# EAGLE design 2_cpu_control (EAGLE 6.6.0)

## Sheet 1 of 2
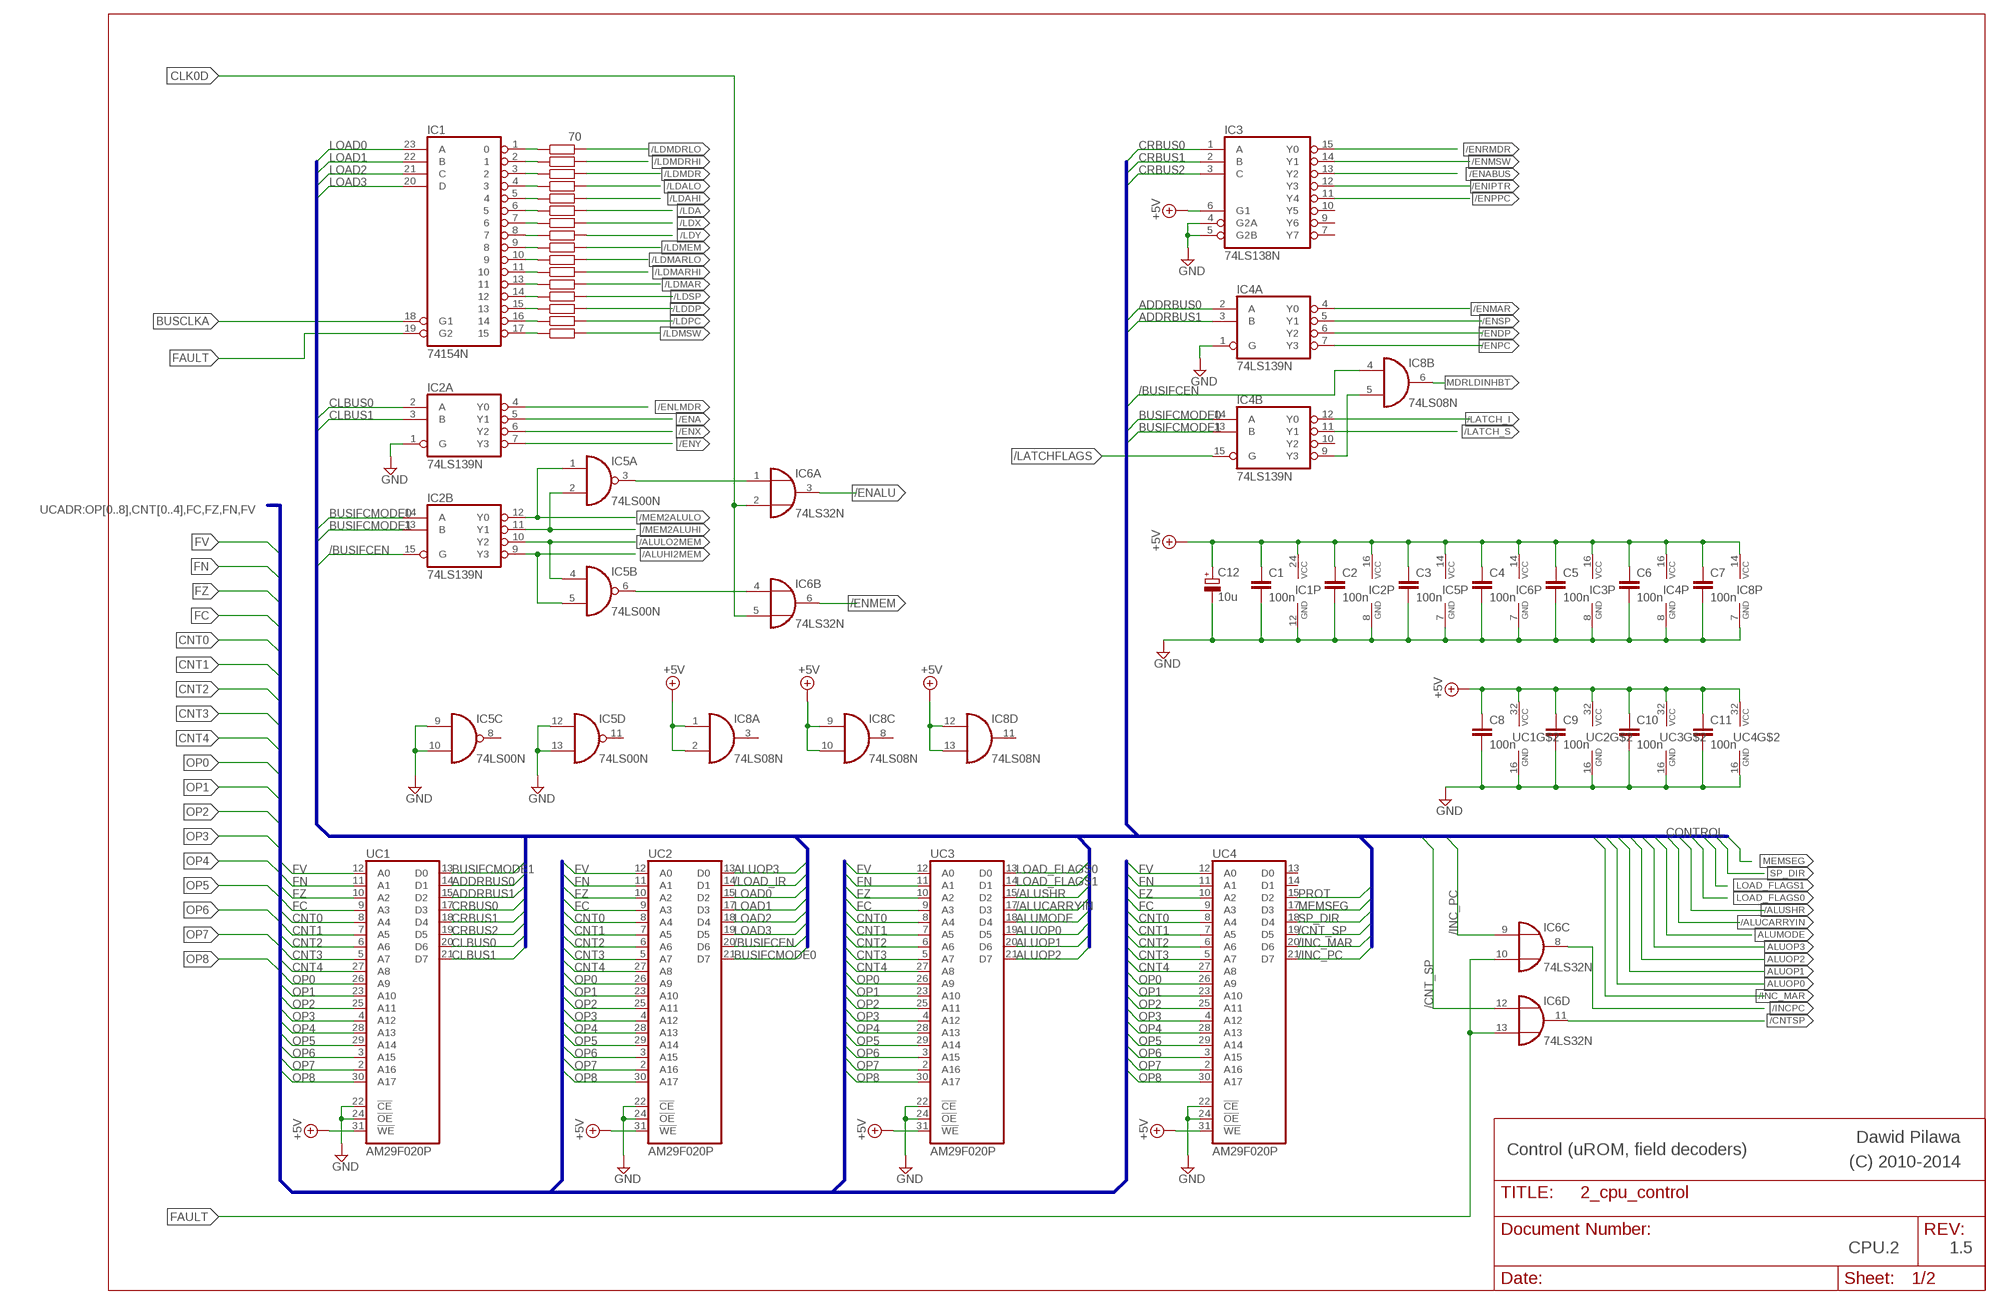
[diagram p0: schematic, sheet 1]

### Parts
C1  100n  C-EU050-024X044  [C050-024X044]
C2  100n  C-EU050-024X044  [C050-024X044]
C3  100n  C-EU050-024X044  [C050-024X044]
C4  100n  C-EU050-024X044  [C050-024X044]
C5  100n  C-EU050-024X044  [C050-024X044]
C6  100n  C-EU050-024X044  [C050-024X044]
C7  100n  C-EU050-024X044  [C050-024X044]
C8  100n  C-EU050-024X044  [C050-024X044]
C9  100n  C-EU050-024X044  [C050-024X044]
C10  100n  C-EU050-024X044  [C050-024X044]
C11  100n  C-EU050-024X044  [C050-024X044]
C12  10u  CPOL-EUE5-6  [E5-6]
IC1  74154N  [DIL24-6]
IC2  74LS139N  [DIL16]
IC3  74LS138N  [DIL16]
IC4  74LS139N  [DIL16]
IC5  74LS00N  [DIL14]
IC6  74LS32N  [DIL14]
IC8  74LS08N  [DIL14]
R1  70  R-EU_0204/7  [0204/7]
R2  R-EU_0204/7  [0204/7]
R3  R-EU_0204/7  [0204/7]
R4  R-EU_0204/7  [0204/7]
R5  R-EU_0204/7  [0204/7]
R6  R-EU_0204/7  [0204/7]
R7  R-EU_0204/7  [0204/7]
R8  R-EU_0204/7  [0204/7]
R9  R-EU_0204/7  [0204/7]
R10  R-EU_0204/7  [0204/7]
R11  R-EU_0204/7  [0204/7]
R12  R-EU_0204/7  [0204/7]
R13  R-EU_0204/7  [0204/7]
R14  R-EU_0204/7  [0204/7]
R15  R-EU_0204/7  [0204/7]
R16  R-EU_0204/7  [0204/7]
UC1  AM29F020P  [DIL32-6]
UC2  AM29F020P  [DIL32-6]
UC3  AM29F020P  [DIL32-6]
UC4  AM29F020P  [DIL32-6]

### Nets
+5V: C1.1 C2.1 C3.1 C4.1 C5.1 C6.1 C7.1 C8.1 C9.1 C10.1 C11.1 C12.+ IC1.24(VCC) IC2.16(P:VCC) IC3.6(G1) IC3.16(VCC) IC4.16(P:VCC) IC5.14(P:VCC) IC6.14(P:VCC) IC8.1(A:I0) IC8.2(A:I1) IC8.9(C:I0) IC8.10(C:I1) IC8.12(D:I0) IC8.13(D:I1) IC8.14(P:VCC) UC1.31(!WE) UC1.32(AVCC) UC2.31(!WE) UC2.32(AVCC) UC3.31(!WE) UC3.32(AVCC) UC4.31(!WE) UC4.32(AVCC) ; also sheet 2
/ALUCARRYIN: UC3.17(D3) ; also sheet 2
/ALUHI2MEM: IC2.9(B:Y3) IC5.5(B:I1) ; also sheet 2
/ALULO2MEM: IC2.10(B:Y2) IC5.4(B:I0) ; also sheet 2
/ALUSHR: UC3.15(D2) ; also sheet 2
/BUSIFCEN: IC2.15(B:G) IC8.4(B:I0) UC2.20(D6) ; also sheet 2
/CNT_SP: IC6.12(D:I0) UC4.19(D5)
/CNTSP: IC6.11(D:O) ; also sheet 2
/ENA: IC2.5(A:Y1) ; also sheet 2
/ENABUS: IC3.13(Y2) ; also sheet 2
/ENALU: IC6.3(A:O) ; also sheet 2
/ENDP: IC4.6(A:Y2) ; also sheet 2
/ENIPTR: IC3.12(Y3) ; also sheet 2
/ENLMDR: IC2.4(A:Y0) ; also sheet 2
/ENMAR: IC4.4(A:Y0) ; also sheet 2
/ENMEM: IC6.6(B:O) ; also sheet 2
/ENMSW: IC3.14(Y1) ; also sheet 2
/ENPC: IC4.7(A:Y3) ; also sheet 2
/ENPPC: IC3.11(Y4) ; also sheet 2
/ENRMDR: IC3.15(Y0) ; also sheet 2
/ENSP: IC4.5(A:Y1) ; also sheet 2
/ENX: IC2.6(A:Y2) ; also sheet 2
/ENY: IC2.7(A:Y3) ; also sheet 2
/INC_MAR: UC4.20(D6) ; also sheet 2
/INC_PC: IC6.9(C:I0) UC4.21(D7)
/INCPC: IC6.8(C:O) ; also sheet 2
/LATCH_I: IC4.12(B:Y0) ; also sheet 2
/LATCH_NONE: IC4.9(B:Y3) IC8.5(B:I1)
/LATCH_S: IC4.11(B:Y1) ; also sheet 2
/LATCHFLAGS: IC4.15(B:G) ; also sheet 2
/LDA: R6.2 ; also sheet 2
/LDAHI: R5.2 ; also sheet 2
/LDALO: R4.2 ; also sheet 2
/LDDP: R14.2 ; also sheet 2
/LDMAR: R12.2 ; also sheet 2
/LDMARHI: R11.2 ; also sheet 2
/LDMARLO: R10.2 ; also sheet 2
/LDMDR: R3.2 ; also sheet 2
/LDMDRHI: R2.2 ; also sheet 2
/LDMDRLO: R1.2 ; also sheet 2
/LDMEM: R9.2 ; also sheet 2
/LDMSW: R16.2 ; also sheet 2
/LDPC: R15.2 ; also sheet 2
/LDSP: R13.2 ; also sheet 2
/LDX: R7.2 ; also sheet 2
/LDY: R8.2 ; also sheet 2
/LOAD_IR: UC2.14(D1) ; also sheet 2
/MEM2ALUHI: IC2.11(B:Y1) IC5.2(A:I1) ; also sheet 2
/MEM2ALULO: IC2.12(B:Y0) IC5.1(A:I0) ; also sheet 2
ADDRBUS0: IC4.2(A:A) UC1.14(D1)
ADDRBUS1: IC4.3(A:B) UC1.15(D2)
ALUMODE: UC3.18(D4) ; also sheet 2
ALUOP0: UC3.19(D5) ; also sheet 2
ALUOP1: UC3.20(D6) ; also sheet 2
ALUOP2: UC3.21(D7) ; also sheet 2
ALUOP3: UC2.13(D0) ; also sheet 2
BUSCLKA: IC1.18(G1) ; also sheet 2
BUSIFCMODE0: IC2.14(B:A) IC4.14(B:A) UC2.21(D7)
BUSIFCMODE1: IC2.13(B:B) IC4.13(B:B) UC1.13(D0)
CLBUS0: IC2.2(A:A) UC1.20(D6)
CLBUS1: IC2.3(A:B) UC1.21(D7)
CLK0D: IC6.2(A:I1) IC6.5(B:I1) ; also sheet 2
CNT0: UC1.8(A4) UC2.8(A4) UC3.8(A4) UC4.8(A4) ; also sheet 2
CNT1: UC1.7(A5) UC2.7(A5) UC3.7(A5) UC4.7(A5) ; also sheet 2
CNT2: UC1.6(A6) UC2.6(A6) UC3.6(A6) UC4.6(A6) ; also sheet 2
CNT3: UC1.5(A7) UC2.5(A7) UC3.5(A7) UC4.5(A7) ; also sheet 2
CNT4: UC1.27(A8) UC2.27(A8) UC3.27(A8) UC4.27(A8) ; also sheet 2
CRBUS0: IC3.1(A) UC1.17(D3)
CRBUS1: IC3.2(B) UC1.18(D4)
CRBUS2: IC3.3(C) UC1.19(D5)
FAULT: IC1.19(G2) IC6.10(C:I1) IC6.13(D:I1) ; also sheet 2
FC: UC1.9(A3) UC2.9(A3) UC3.9(A3) UC4.9(A3) ; also sheet 2
FN: UC1.11(A1) UC2.11(A1) UC3.11(A1) UC4.11(A1) ; also sheet 2
FV: UC1.12(A0) UC2.12(A0) UC3.12(A0) UC4.12(A0) ; also sheet 2
FZ: UC1.10(A2) UC2.10(A2) UC3.10(A2) UC4.10(A2) ; also sheet 2
GND: C1.2 C2.2 C3.2 C4.2 C5.2 C6.2 C7.2 C8.2 C9.2 C10.2 C11.2 C12.- IC1.12(GND) IC2.1(A:G) IC2.8(P:GND) IC3.4(G2A) IC3.5(G2B) IC3.8(GND) IC4.1(A:G) IC4.8(P:GND) IC5.7(P:GND) IC5.9(C:I0) IC5.10(C:I1) IC5.12(D:I0) IC5.13(D:I1) IC6.7(P:GND) IC8.7(P:GND) UC1.16(AGND) UC1.22(!CE) UC1.24(!OE) UC2.16(AGND) UC2.22(!CE) UC2.24(!OE) UC3.16(AGND) UC3.22(!CE) UC3.24(!OE) UC4.16(AGND) UC4.22(!CE) UC4.24(!OE) ; also sheet 2
LOAD0: IC1.23(A) UC2.15(D2)
LOAD1: IC1.22(B) UC2.17(D3)
LOAD2: IC1.21(C) UC2.18(D4)
LOAD3: IC1.20(D) UC2.19(D5)
LOAD_FLAGS0: UC3.13(D0) ; also sheet 2
LOAD_FLAGS1: UC3.14(D1) ; also sheet 2
MDRLDINHBT: IC8.6(B:O) ; also sheet 2
MEMSEG: UC4.17(D3) ; also sheet 2
N$1: IC1.16 R15.1
N$8: IC5.3(A:O) IC6.1(A:I0)
N$15: IC5.6(B:O) IC6.4(B:I0)
N$31: IC1.1 R1.1
N$33: IC1.2 R2.1
N$34: IC1.3 R3.1
N$35: IC1.4 R4.1
N$36: IC1.5 R5.1
N$37: IC1.6 R6.1
N$38: IC1.7 R7.1
N$39: IC1.8 R8.1
N$40: IC1.9 R9.1
N$41: IC1.10 R10.1
N$42: IC1.11 R11.1
N$43: IC1.13 R12.1
N$44: IC1.14 R13.1
N$45: IC1.15 R14.1
N$56: IC1.17 R16.1
OP0: UC1.26(A9) UC2.26(A9) UC3.26(A9) UC4.26(A9) ; also sheet 2
OP1: UC1.23(A10) UC2.23(A10) UC3.23(A10) UC4.23(A10) ; also sheet 2
OP2: UC1.25(A11) UC2.25(A11) UC3.25(A11) UC4.25(A11) ; also sheet 2
OP3: UC1.4(A12) UC2.4(A12) UC3.4(A12) UC4.4(A12) ; also sheet 2
OP4: UC1.28(A13) UC2.28(A13) UC3.28(A13) UC4.28(A13) ; also sheet 2
OP5: UC1.29(A14) UC2.29(A14) UC3.29(A14) UC4.29(A14) ; also sheet 2
OP6: UC1.3(A15) UC2.3(A15) UC3.3(A15) UC4.3(A15) ; also sheet 2
OP7: UC1.2(A16) UC2.2(A16) UC3.2(A16) UC4.2(A16) ; also sheet 2
OP8: UC1.30(A17) UC2.30(A17) UC3.30(A17) UC4.30(A17) ; also sheet 2
PROT: UC4.15(D2) ; also sheet 2
SP_DIR: UC4.18(D4) ; also sheet 2
Unconnected: IC3.7(Y7) IC3.9(Y6) IC3.10(Y5) IC4.10(B:Y2) IC5.8(C:O) IC5.11(D:O) IC8.3(A:O) IC8.8(C:O) IC8.11(D:O) UC4.13(D0) UC4.14(D1)

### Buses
UCADR:OP[0..8],CNT[0..4],FC,FZ,FN,FV
UCODE:CLBUS[0..1],CRBUS[0..2],ADDRBUS[0..1],BUSIFCMODE[0..1],/BUSIFCEN,LOAD[0..3],/LOAD_IR,ALUOP[0..3],ALUMODE,/ALUCARRYIN,/ALUSHR,LOAD_FLAGS[0..1],/INC_PC,/INC_MAR,/CNT_SP,SP_DIR,MEMSEG,PROT,NC[0..1],NEXTOP

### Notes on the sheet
- CONTROL
- Dawid Pilawa
- Control (uROM, field decoders) | (C) 2010-2014
- CPU.2 | 1.5

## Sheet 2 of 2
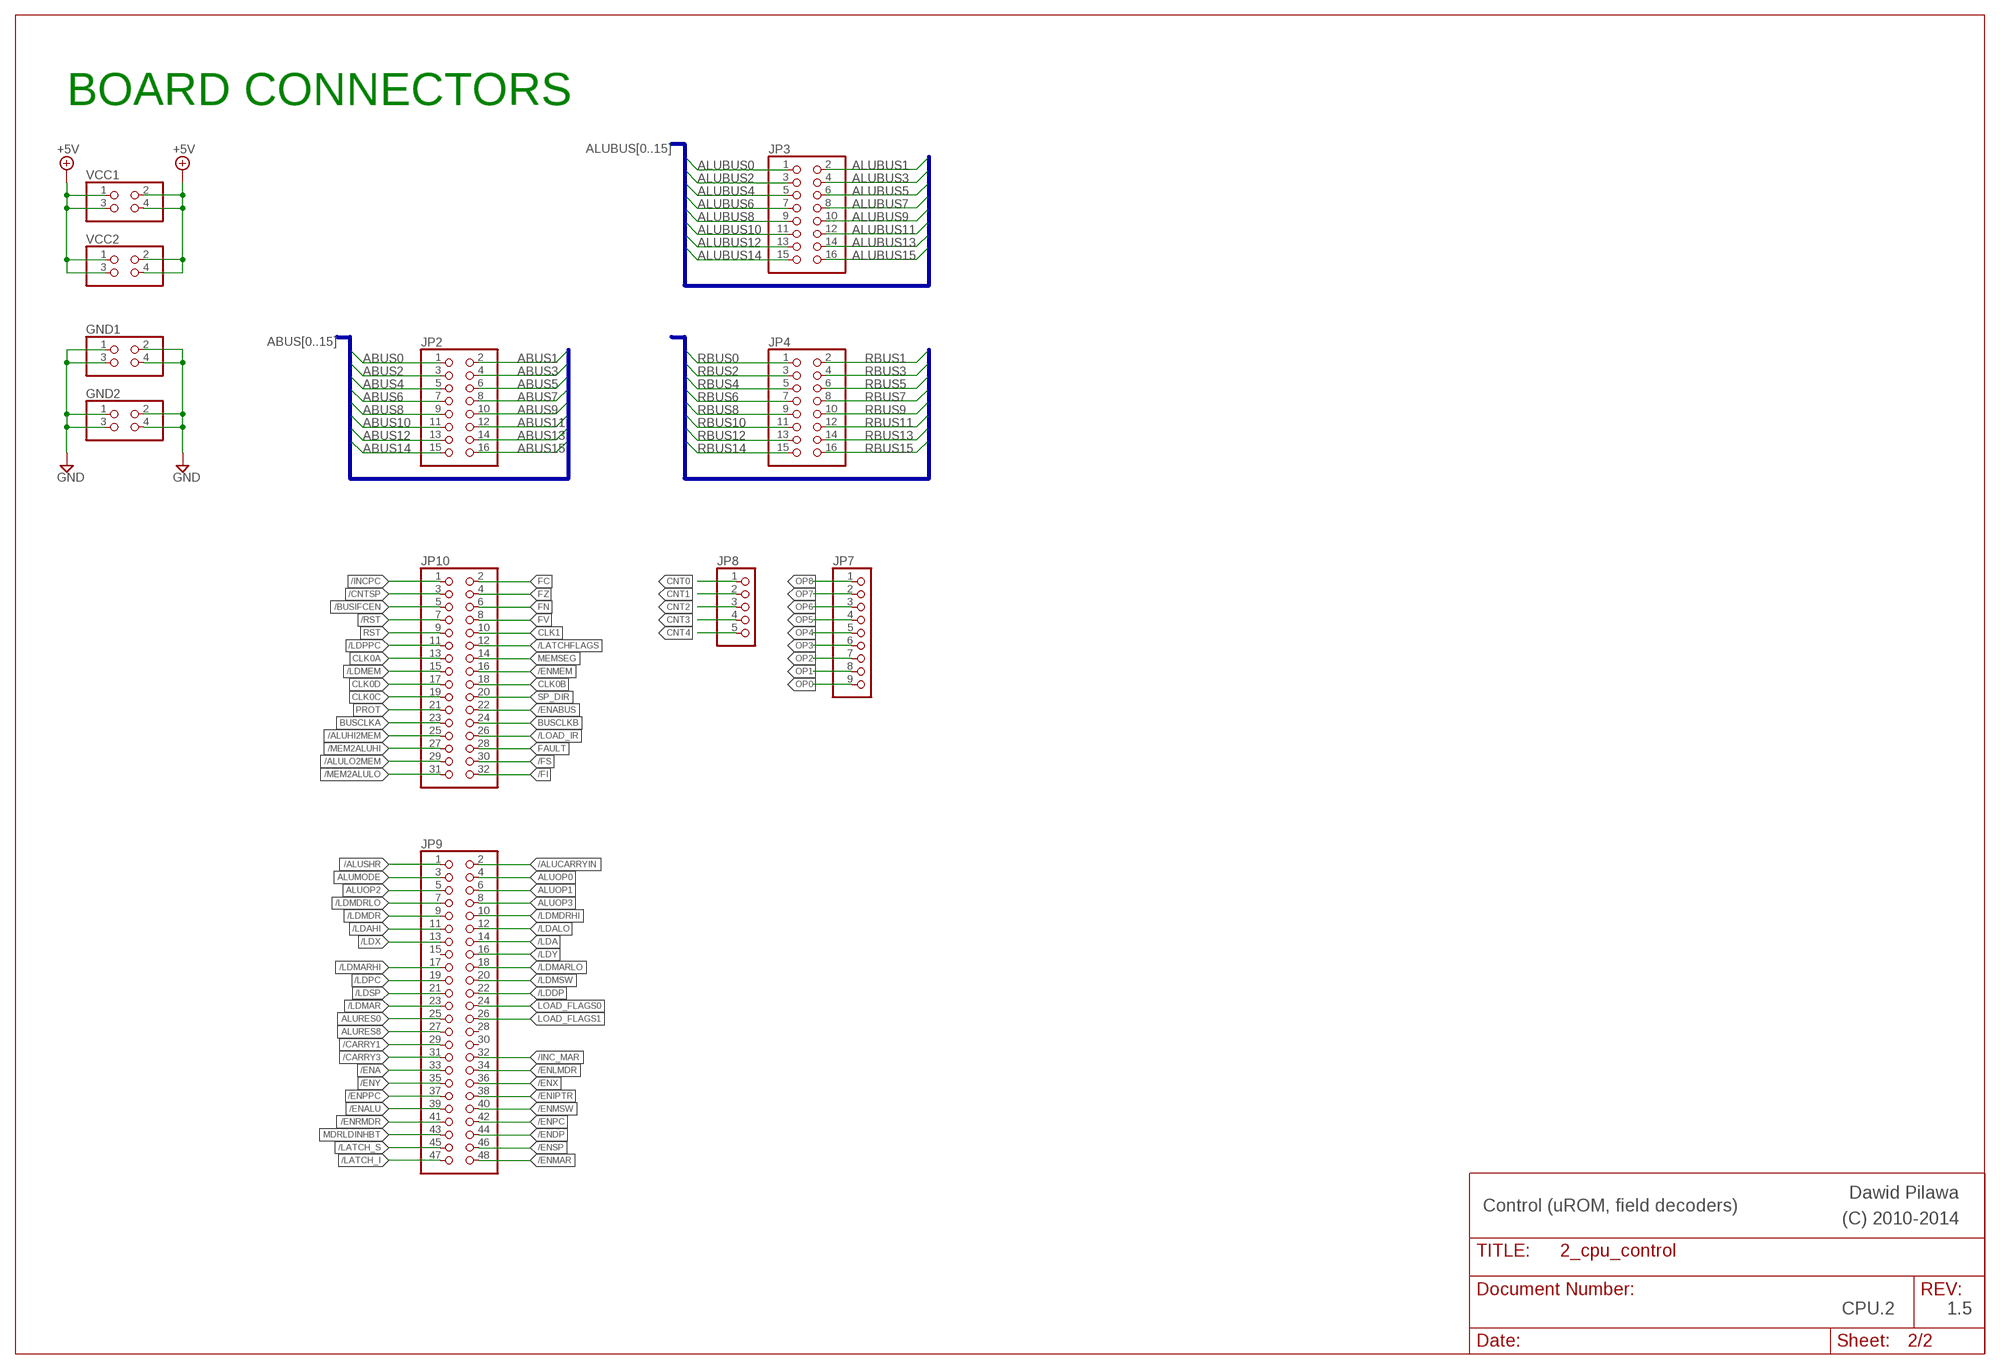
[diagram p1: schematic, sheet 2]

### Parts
GND1  PINHD-2X2  [2X02]
GND2  PINHD-2X2  [2X02]
JP2  PINHD-2X8  [2X08]
JP3  PINHD-2X8  [2X08]
JP4  PINHD-2X8  [2X08]
JP7  PINHD-1X9  [1X09]
JP8  PINHD-1X5  [1X05]
JP9  PINHD-2X24  [2X24]
JP10  PINHD-2X16  [2X16]
VCC1  PINHD-2X2  [2X02]
VCC2  PINHD-2X2  [2X02]

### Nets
+5V: VCC1.1 VCC1.2 VCC1.3 VCC1.4 VCC2.1 VCC2.2 VCC2.3 VCC2.4 ; also sheet 1
/ALUCARRYIN: JP9.2 ; also sheet 1
/ALUHI2MEM: JP10.25 ; also sheet 1
/ALULO2MEM: JP10.29 ; also sheet 1
/ALUSHR: JP9.1 ; also sheet 1
/BUSIFCEN: JP10.5 ; also sheet 1
/CARRY1: JP9.29
/CARRY3: JP9.31
/CNTSP: JP10.3 ; also sheet 1
/ENA: JP9.33 ; also sheet 1
/ENABUS: JP10.22 ; also sheet 1
/ENALU: JP9.39 ; also sheet 1
/ENDP: JP9.44 ; also sheet 1
/ENIPTR: JP9.38 ; also sheet 1
/ENLMDR: JP9.34 ; also sheet 1
/ENMAR: JP9.48 ; also sheet 1
/ENMEM: JP10.16 ; also sheet 1
/ENMSW: JP9.40 ; also sheet 1
/ENPC: JP9.42 ; also sheet 1
/ENPPC: JP9.37 ; also sheet 1
/ENRMDR: JP9.41 ; also sheet 1
/ENSP: JP9.46 ; also sheet 1
/ENX: JP9.36 ; also sheet 1
/ENY: JP9.35 ; also sheet 1
/FI: JP10.32
/FS: JP10.30
/INC_MAR: JP9.32 ; also sheet 1
/INCPC: JP10.1 ; also sheet 1
/LATCH_I: JP9.47 ; also sheet 1
/LATCH_S: JP9.45 ; also sheet 1
/LATCHFLAGS: JP10.12 ; also sheet 1
/LDA: JP9.14 ; also sheet 1
/LDAHI: JP9.11 ; also sheet 1
/LDALO: JP9.12 ; also sheet 1
/LDDP: JP9.22 ; also sheet 1
/LDMAR: JP9.23 ; also sheet 1
/LDMARHI: JP9.17 ; also sheet 1
/LDMARLO: JP9.18 ; also sheet 1
/LDMDR: JP9.9 ; also sheet 1
/LDMDRHI: JP9.10 ; also sheet 1
/LDMDRLO: JP9.7 ; also sheet 1
/LDMEM: JP10.15 ; also sheet 1
/LDMSW: JP9.20 ; also sheet 1
/LDPC: JP9.19 ; also sheet 1
/LDPPC: JP10.11
/LDSP: JP9.21 ; also sheet 1
/LDX: JP9.13 ; also sheet 1
/LDY: JP9.16 ; also sheet 1
/LOAD_IR: JP10.26 ; also sheet 1
/MEM2ALUHI: JP10.27 ; also sheet 1
/MEM2ALULO: JP10.31 ; also sheet 1
/RST: JP10.7
ABUS0: JP2.1
ABUS1: JP2.2
ABUS2: JP2.3
ABUS3: JP2.4
ABUS4: JP2.5
ABUS5: JP2.6
ABUS6: JP2.7
ABUS7: JP2.8
ABUS8: JP2.9
ABUS9: JP2.10
ABUS10: JP2.11
ABUS11: JP2.12
ABUS12: JP2.13
ABUS13: JP2.14
ABUS14: JP2.15
ABUS15: JP2.16
ALUBUS0: JP3.1
ALUBUS1: JP3.2
ALUBUS2: JP3.3
ALUBUS3: JP3.4
ALUBUS4: JP3.5
ALUBUS5: JP3.6
ALUBUS6: JP3.7
ALUBUS7: JP3.8
ALUBUS8: JP3.9
ALUBUS9: JP3.10
ALUBUS10: JP3.11
ALUBUS11: JP3.12
ALUBUS12: JP3.13
ALUBUS13: JP3.14
ALUBUS14: JP3.15
ALUBUS15: JP3.16
ALUMODE: JP9.3 ; also sheet 1
ALUOP0: JP9.4 ; also sheet 1
ALUOP1: JP9.6 ; also sheet 1
ALUOP2: JP9.5 ; also sheet 1
ALUOP3: JP9.8 ; also sheet 1
ALURES0: JP9.25
ALURES8: JP9.27
BUSCLKA: JP10.23 ; also sheet 1
BUSCLKB: JP10.24
CLK0A: JP10.13
CLK0B: JP10.18
CLK0C: JP10.19
CLK0D: JP10.17 ; also sheet 1
CLK1: JP10.10
CNT0: JP8.1 ; also sheet 1
CNT1: JP8.2 ; also sheet 1
CNT2: JP8.3 ; also sheet 1
CNT3: JP8.4 ; also sheet 1
CNT4: JP8.5 ; also sheet 1
FAULT: JP10.28 ; also sheet 1
FC: JP10.2 ; also sheet 1
FN: JP10.6 ; also sheet 1
FV: JP10.8 ; also sheet 1
FZ: JP10.4 ; also sheet 1
GND: GND1.1 GND1.2 GND1.3 GND1.4 GND2.1 GND2.2 GND2.3 GND2.4 ; also sheet 1
LOAD_FLAGS0: JP9.24 ; also sheet 1
LOAD_FLAGS1: JP9.26 ; also sheet 1
MDRLDINHBT: JP9.43 ; also sheet 1
MEMSEG: JP10.14 ; also sheet 1
OP0: JP7.9 ; also sheet 1
OP1: JP7.8 ; also sheet 1
OP2: JP7.7 ; also sheet 1
OP3: JP7.6 ; also sheet 1
OP4: JP7.5 ; also sheet 1
OP5: JP7.4 ; also sheet 1
OP6: JP7.3 ; also sheet 1
OP7: JP7.2 ; also sheet 1
OP8: JP7.1 ; also sheet 1
PROT: JP10.21 ; also sheet 1
RBUS0: JP4.1
RBUS1: JP4.2
RBUS2: JP4.3
RBUS3: JP4.4
RBUS4: JP4.5
RBUS5: JP4.6
RBUS6: JP4.7
RBUS7: JP4.8
RBUS8: JP4.9
RBUS9: JP4.10
RBUS10: JP4.11
RBUS11: JP4.12
RBUS12: JP4.13
RBUS13: JP4.14
RBUS14: JP4.15
RBUS15: JP4.16
RST: JP10.9
SP_DIR: JP10.20 ; also sheet 1
Unconnected: JP9.15 JP9.28 JP9.30

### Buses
ALUBUS[0..15]
RBUS[0..15]
ABUS[0..15]

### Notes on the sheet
- BOARD CONNECTORS
- Dawid Pilawa
- Control (uROM, field decoders) | (C) 2010-2014
- CPU.2 | 1.5

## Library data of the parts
C1-C11 = rcl:C-EU: CAPACITOR, European symbol
C12 = rcl:CPOL-EU: POLARIZED CAPACITOR, European symbol
GND1 GND2 VCC1 VCC2 = pinhead:PINHD-2X2: PIN HEADER
IC1 = 74xx-eu:74*154: 4-line to 16-line data SELECTOR/MULTIPLEXER
IC2 IC4 = 74xx-eu:74*139: Dual 2-line to 4-line DECODER/DEMULTIPLEXER
IC3 = 74xx-eu:74*138: 3-line to 8-line DECODER/DEMULTIPLEXER
IC5 = 74xx-eu:74*00: Quad 2-input NAND gate
IC6 = 74xx-eu:74*32: Quad 2-input OR gate
IC8 = 74xx-eu:74*08: Quad 2-input AND gate
JP2-JP4 = pinhead:PINHD-2X8: PIN HEADER
JP7 = pinhead:PINHD-1X9: PIN HEADER
JP8 = pinhead:PINHD-1X5: PIN HEADER
JP9 = pinhead:PINHD-2X24: PIN HEADER
JP10 = pinhead:PINHD-2X16: PIN HEADER
R1-R16 = rcl:R-EU_: RESISTOR, European symbol
UC1-UC4 = am29-memory:AM29F020P: 20F020 - 256kB FLASH

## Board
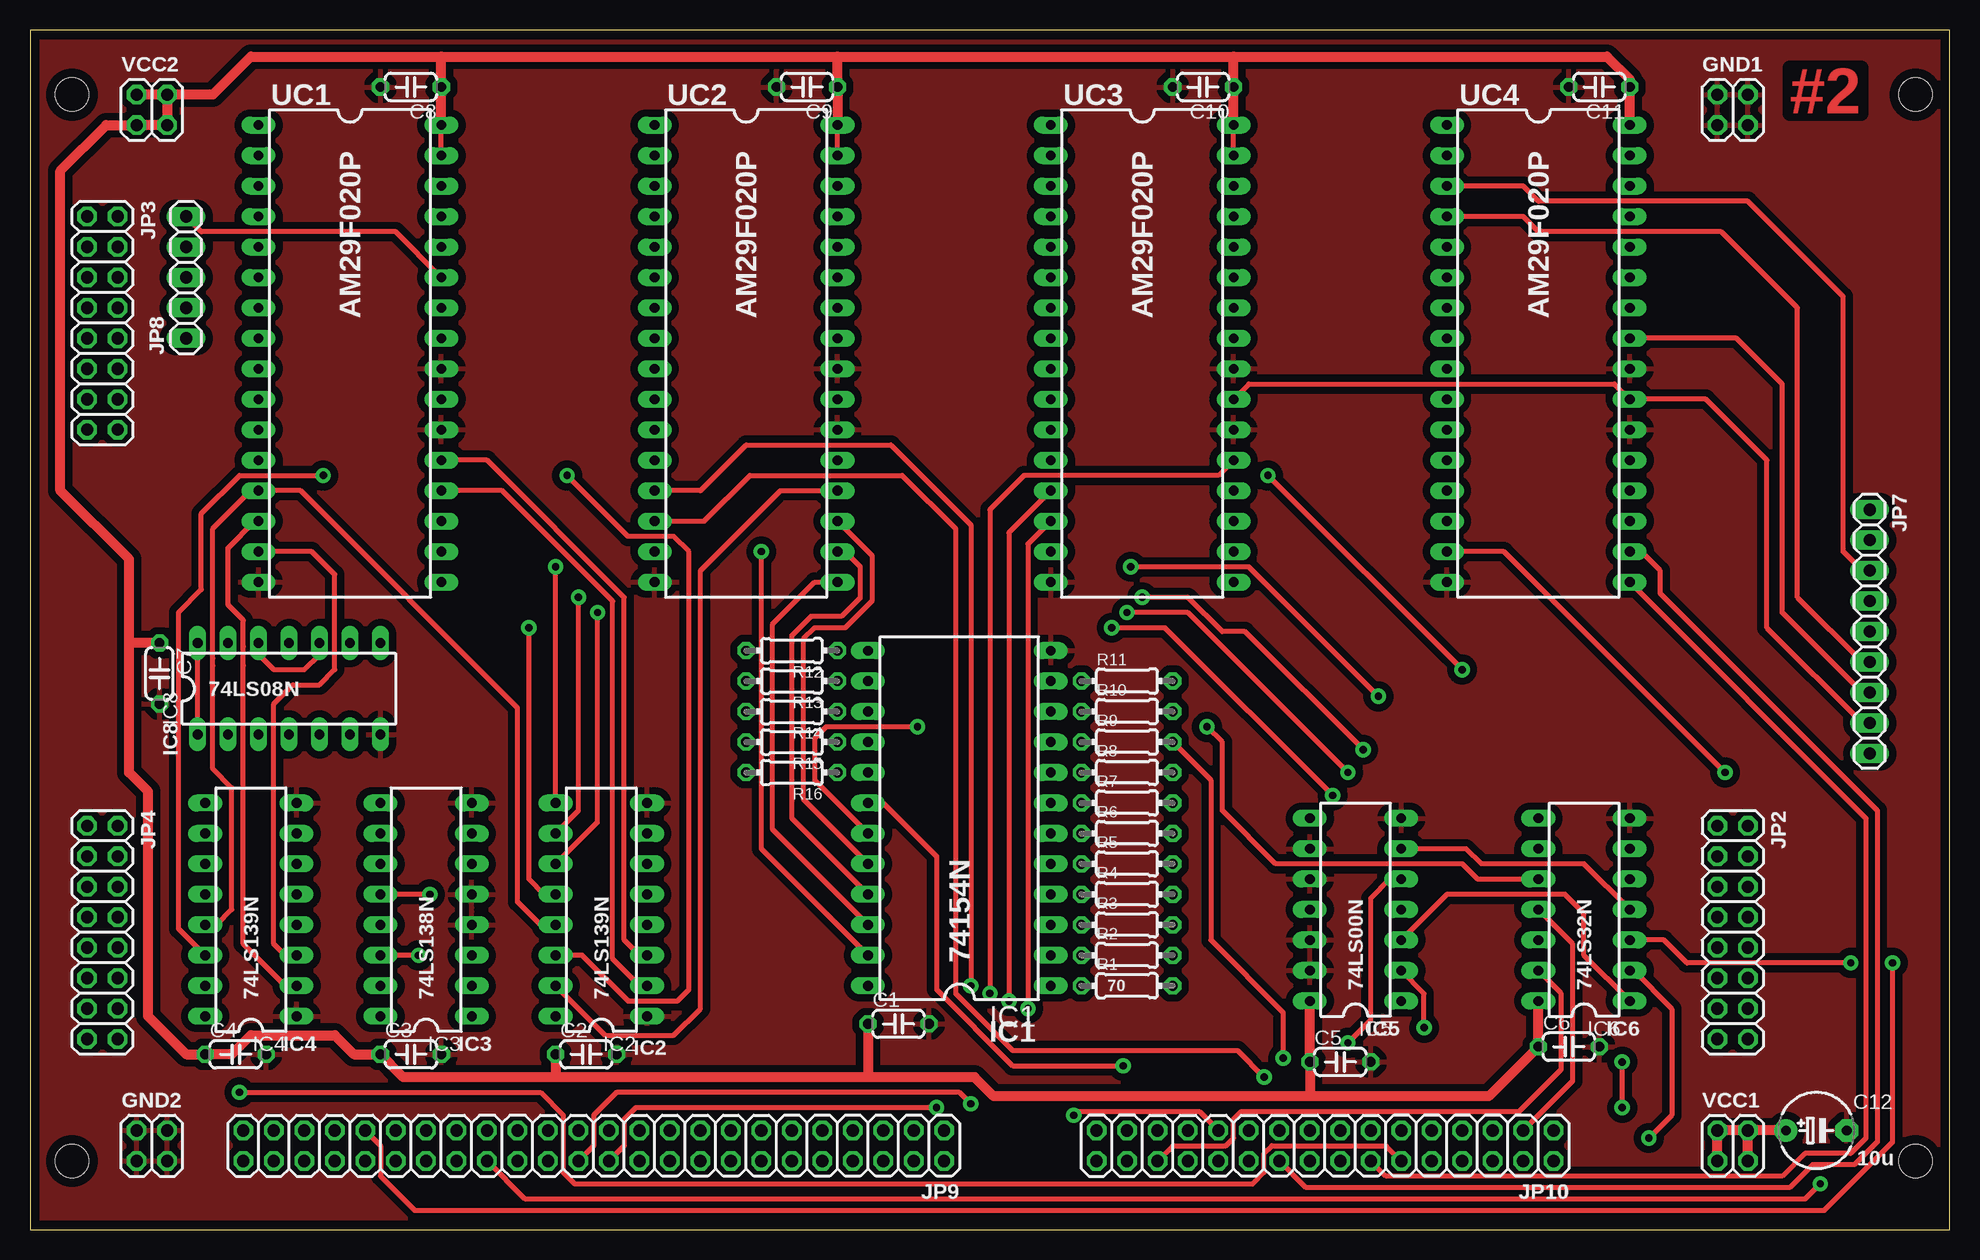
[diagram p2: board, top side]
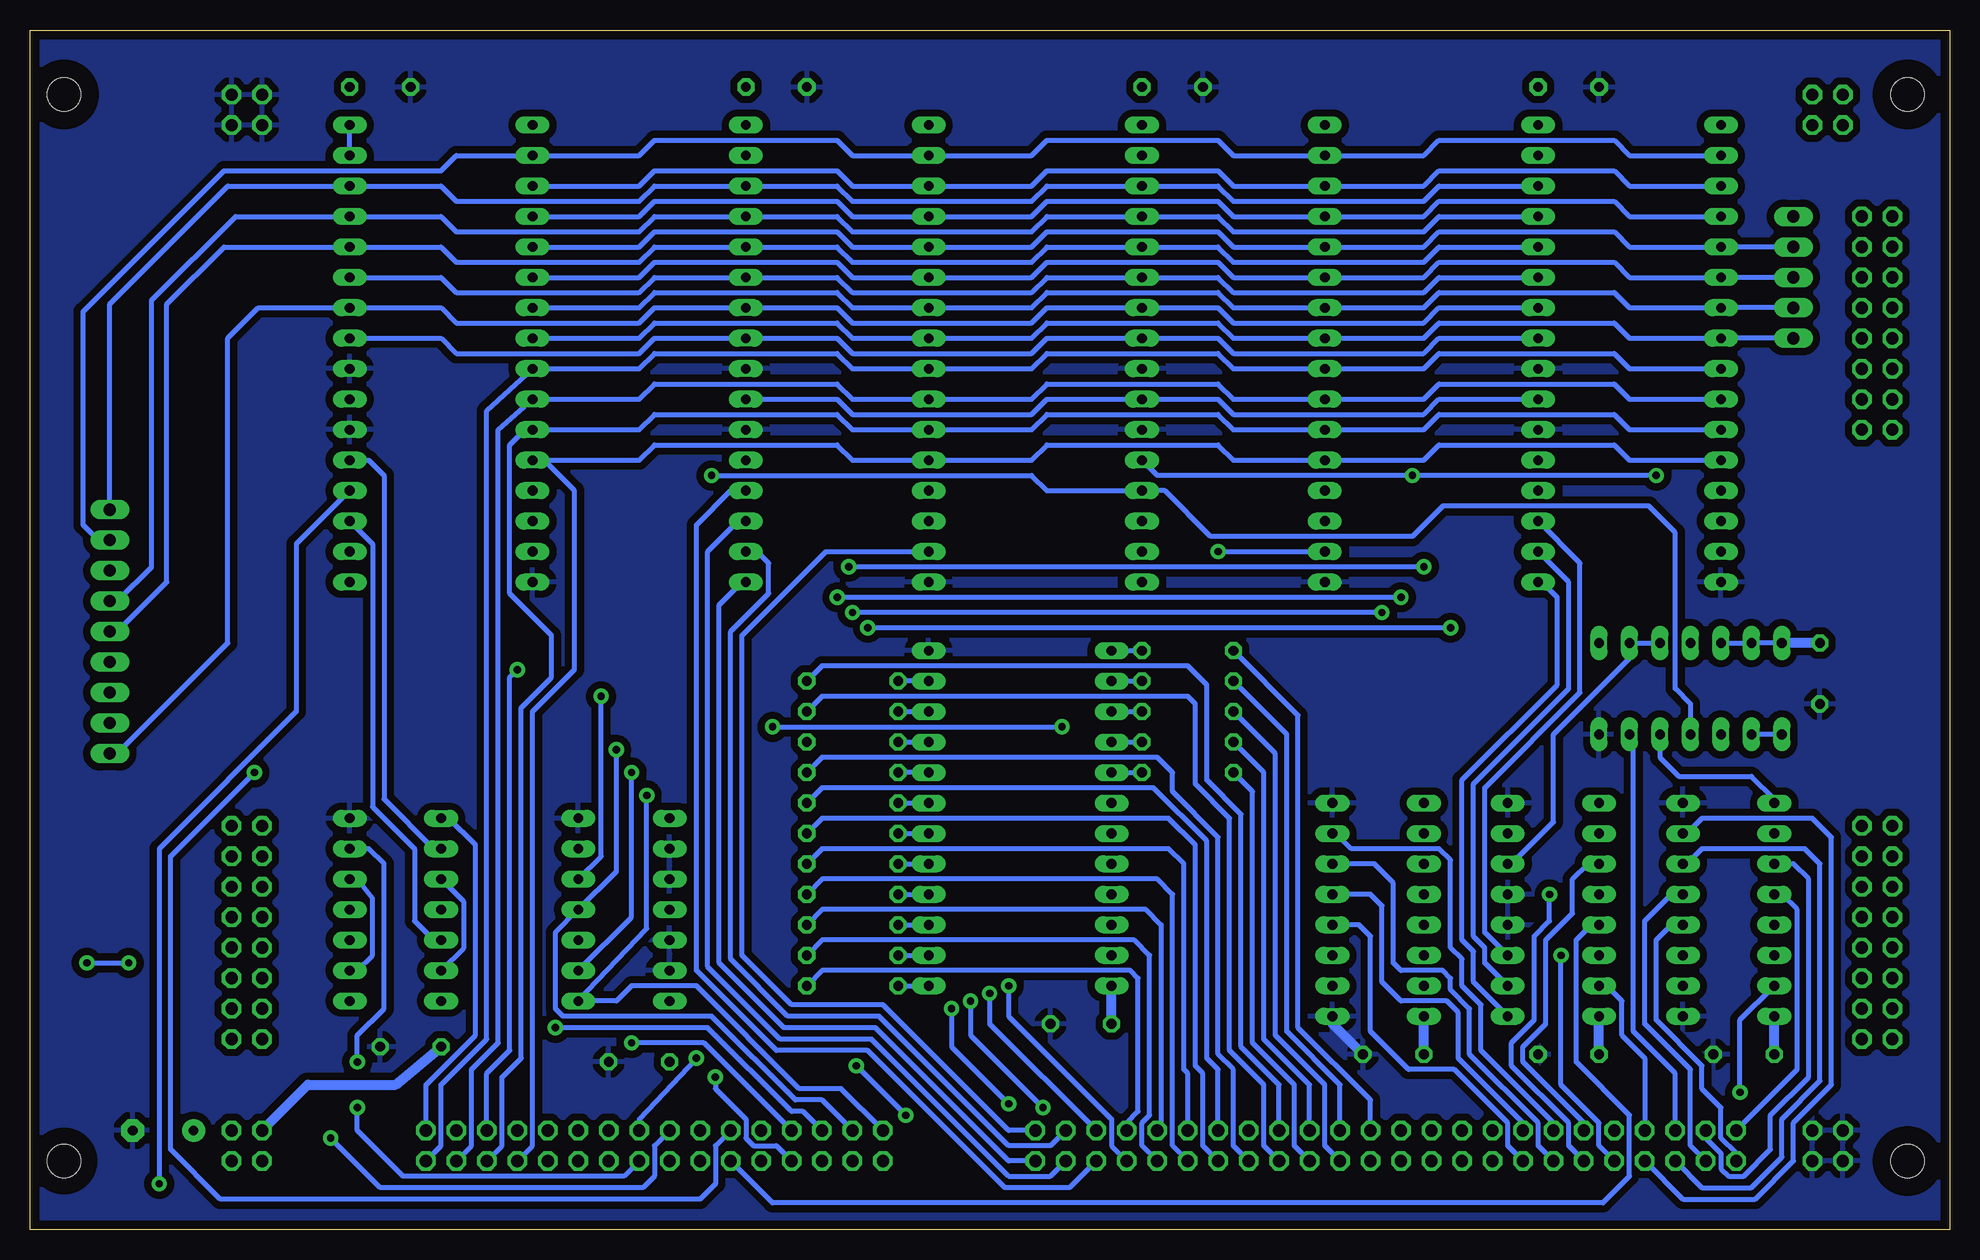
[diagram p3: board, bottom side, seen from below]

Size 160 x 100 mm. Coordinates in mm from the lower left corner, seen from the top.
Outline: 0,0 160,0 160,100 0,100 0,0
Copper layers (1*16): Top 0.035mm / dielectric 1.5mm / Bottom 0.035mm
Design rules "homebrew_pcb": minimum track width 16mil, minimum drill 24mil, track to track 16mil, track to pad 10mil, pad to pad 10mil, via to via 10mil, smd to smd 8mil, copper to edge 30mil, drill to drill 10mil, minimum pad ring 12mil, minimum via ring 12mil, stop-mask expansion 4mil, vias tented up to drill 0mil, thermal gap 24mil
Holes 2.79 mm at 3.49,94.61 157.16,94.61 157.16,5.71 3.49,5.71
bRestrict: area 1.2,3.4 to 5.8,8; area 155,3.6 to 159.3,7.9; area 154.9,92.3 to 159.4,96.9; area 1.2,92.3 to 5.8,96.9
vRestrict: area 155,3.6 to 159.3,7.9; area 154.9,92.3 to 159.4,96.9; area 1.2,3.4 to 5.8,8; area 1.2,92.3 to 5.8,96.9

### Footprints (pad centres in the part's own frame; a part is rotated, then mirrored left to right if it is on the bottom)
C050-024X044 = drill 0.813 octagon: 1 -2.54,0; 2 2.54,0
E5-6 = drill 0.813 pad 1.905: + -2.54,0 | drill 0.813 pad 1.905 octagon: - 2.54,0
2X02 = drill 1.016 octagon: 1 -1.27,-1.27; 2 -1.27,1.27; 3 1.27,-1.27; 4 1.27,1.27
DIL24-6 = drill 0.813 long: 1 -13.97,-7.62; 2 -11.43,-7.62; 3 -8.89,-7.62; 4 -6.35,-7.62; 5 -3.81,-7.62; 6 -1.27,-7.62; 7 1.27,-7.62; 8 3.81,-7.62; 9 6.35,-7.62; 10 8.89,-7.62; 11 11.43,-7.62; 12 13.97,-7.62; 13 13.97,7.62; 14 11.43,7.62; 15 8.89,7.62; 16 6.35,7.62; 17 3.81,7.62; 18 1.27,7.62; 19 -1.27,7.62; 20 -3.81,7.62; 21 -6.35,7.62; 22 -8.89,7.62; 23 -11.43,7.62; 24 -13.97,7.62
DIL16 = drill 0.813 long: 1 -8.89,-3.81; 2 -6.35,-3.81; 3 -3.81,-3.81; 4 -1.27,-3.81; 5 1.27,-3.81; 6 3.81,-3.81; 7 6.35,-3.81; 8 8.89,-3.81; 9 8.89,3.81; 10 6.35,3.81; 11 3.81,3.81; 12 1.27,3.81; 13 -1.27,3.81; 14 -3.81,3.81; 15 -6.35,3.81; 16 -8.89,3.81
DIL14 = drill 0.813 long: 1 -7.62,-3.81; 2 -5.08,-3.81; 3 -2.54,-3.81; 4 0,-3.81; 5 2.54,-3.81; 6 5.08,-3.81; 7 7.62,-3.81; 8 7.62,3.81; 9 5.08,3.81; 10 2.54,3.81; 11 0,3.81; 12 -2.54,3.81; 13 -5.08,3.81; 14 -7.62,3.81
2X08 = drill 1.016 octagon: 1 -8.89,-1.27; 2 -8.89,1.27; 3 -6.35,-1.27; 4 -6.35,1.27; 5 -3.81,-1.27; 6 -3.81,1.27; 7 -1.27,-1.27; 8 -1.27,1.27; 9 1.27,-1.27; 10 1.27,1.27; 11 3.81,-1.27; 12 3.81,1.27; 13 6.35,-1.27; 14 6.35,1.27; 15 8.89,-1.27; 16 8.89,1.27
1X09 = drill 1.016 long: 1 -10.16,0; 2 -7.62,0; 3 -5.08,0; 4 -2.54,0; 5 0,0; 6 2.54,0; 7 5.08,0; 8 7.62,0; 9 10.16,0
1X05 = drill 1.016 long: 1 -5.08,0; 2 -2.54,0; 3 0,0; 4 2.54,0; 5 5.08,0
2X24 = drill 1.016 octagon: 1 -27.94,-1.27; 2 -27.94,1.27; 3 -25.4,-1.27; 4 -25.4,1.27; 5 -22.86,-1.27; 6 -22.86,1.27; 7 -20.32,-1.27; 8 -20.32,1.27; 9 -17.78,-1.27; 10 -17.78,1.27; 11 -15.24,-1.27; 12 -15.24,1.27; 13 -12.7,-1.27; 14 -12.7,1.27; 15 -10.16,-1.27; 16 -10.16,1.27; 17 -7.62,-1.27; 18 -7.62,1.27; 19 -5.08,-1.27; 20 -5.08,1.27; 21 -2.54,-1.27; 22 -2.54,1.27; 23 0,-1.27; 24 0,1.27; 25 2.54,-1.27; 26 2.54,1.27; 27 5.08,-1.27; 28 5.08,1.27; 29 7.62,-1.27; 30 7.62,1.27; 31 10.16,-1.27; 32 10.16,1.27; 33 12.7,-1.27; 34 12.7,1.27; 35 15.24,-1.27; 36 15.24,1.27; 37 17.78,-1.27; 38 17.78,1.27; 39 20.32,-1.27; 40 20.32,1.27; 41 22.86,-1.27; 42 22.86,1.27; 43 25.4,-1.27; 44 25.4,1.27; 45 27.94,-1.27; 46 27.94,1.27; 47 30.48,-1.27; 48 30.48,1.27
2X16 = drill 1.016 octagon: 1 -19.05,-1.27; 2 -19.05,1.27; 3 -16.51,-1.27; 4 -16.51,1.27; 5 -13.97,-1.27; 6 -13.97,1.27; 7 -11.43,-1.27; 8 -11.43,1.27; 9 -8.89,-1.27; 10 -8.89,1.27; 11 -6.35,-1.27; 12 -6.35,1.27; 13 -3.81,-1.27; 14 -3.81,1.27; 15 -1.27,-1.27; 16 -1.27,1.27; 17 1.27,-1.27; 18 1.27,1.27; 19 3.81,-1.27; 20 3.81,1.27; 21 6.35,-1.27; 22 6.35,1.27; 23 8.89,-1.27; 24 8.89,1.27; 25 11.43,-1.27; 26 11.43,1.27; 27 13.97,-1.27; 28 13.97,1.27; 29 16.51,-1.27; 30 16.51,1.27; 31 19.05,-1.27; 32 19.05,1.27
0204/7 = drill 0.813 octagon: 1 -3.81,0; 2 3.81,0
DIL32-6 = drill 0.813 long: 1 -17.78,-7.62; 2 -15.24,-7.62; 3 -12.7,-7.62; 4 -10.16,-7.62; 5 -7.62,-7.62; 6 -5.08,-7.62; 7 -2.54,-7.62; 8 0,-7.62; 9 2.54,-7.62; 10 5.08,-7.62; 11 7.62,-7.62; 12 10.16,-7.62; 13 12.7,-7.62; 14 15.24,-7.62; 15 17.78,-7.62; 16 20.32,-7.62; 17 20.32,7.62; 18 17.78,7.62; 19 15.24,7.62; 20 12.7,7.62; 21 10.16,7.62; 22 7.62,7.62; 23 5.08,7.62; 24 2.54,7.62; 25 0,7.62; 26 -2.54,7.62; 27 -5.08,7.62; 28 -7.62,7.62; 29 -10.16,7.62; 30 -12.7,7.62; 31 -15.24,7.62; 32 -17.78,7.62

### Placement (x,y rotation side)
C1  72.39,17.14 0 top
C2  46.35,14.61 0 top
C3  31.75,14.61 0 top
C4  17.14,14.61 0 top
C5  109.22,13.97 0 top
C6  128.27,15.24 0 top
C7  10.79,46.35 270 top
C8  31.75,95.25 180 top
C9  64.77,95.25 180 top
C10  97.79,95.25 180 top
C11  130.81,95.25 180 top
C12  148.91,8.26 0 top
GND1  141.92,93.34 0 top
GND2  10.16,6.99 0 top
IC1  77.47,34.29 90 top
IC2  47.62,26.67 90 top
IC3  33.02,26.67 90 top
IC4  18.41,26.67 90 top
IC5  110.49,26.67 90 top
IC6  129.54,26.67 90 top
IC8  21.59,45.09 0 top
JP2  141.92,24.77 270 top
JP3  6.03,75.56 270 top
JP4  6.03,24.77 270 top
JP7  153.35,49.85 270 top
JP8  13.02,79.38 90 top
JP9  48.26,6.99 180 top
JP10  107.95,6.99 180 top
R1  91.44,20.32 0 top
R2  91.44,22.86 0 top
R3  91.44,25.4 0 top
R4  91.44,27.94 0 top
R5  91.44,30.48 0 top
R6  91.44,33.02 0 top
R7  91.44,35.56 0 top
R8  91.44,38.1 0 top
R9  91.44,40.64 0 top
R10  91.44,43.18 0 top
R11  91.44,45.72 0 top
R12  63.5,48.26 180 top
R13  63.5,45.72 180 top
R14  63.5,43.18 180 top
R15  63.5,40.64 180 top
R16  63.5,38.1 180 top
UC1  26.67,74.3 270 top
UC2  59.69,74.3 270 top
UC3  92.71,74.3 270 top
UC4  125.73,74.3 270 top
VCC1  141.92,6.99 0 top
VCC2  10.16,93.34 0 top

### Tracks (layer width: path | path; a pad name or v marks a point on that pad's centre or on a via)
+5V
  Top 0.406: IC8.1 IC8.14 | UC3.31 UC3.32 | UC2.31 UC2.32 | UC1.31 UC1.32 | IC8.12 19.05,47.94 20.32,46.67 22.86,46.67 24.13,47.94 IC8.10
  Top 0.813: C12.+ VCC1.4 | VCC1.3 VCC1.4 | VCC1.4 VCC1.2 VCC1.1 | 106.68,11.11 121.6,11.11 C6.1 IC6.14 | 106.68,11.11 80.33,11.11 78.74,12.7 69.85,12.7 | 69.85,12.7 43.81,12.7 | 43.81,12.7 31.11,12.7 C3.1 26.99,14.61 25.4,16.19 18.41,16.19 16.83,14.61 C4.1 13.02,14.61 9.84,17.78 9.84,36.51 8.26,38.1 8.26,48.9 | 8.26,48.9 8.26,55.88 2.54,61.59 2.54,88.27 6.35,92.08 VCC2.1 VCC2.3 VCC2.4 | 34.29,97.79 18.41,97.79 15.24,94.61 VCC2.4 | 34.29,97.79 67.31,97.79 | 67.31,97.79 100.33,97.79 | 100.33,97.79 131.44,97.79 133.35,95.89 C11.1 UC4.32 | 106.68,11.11 C5.1 IC5.14 | C2.1 43.81,12.7 | C7.1 8.26,48.9 | VCC2.4 VCC2.2 | 34.29,97.79 C8.1 UC1.32 | 67.31,97.79 C9.1 UC2.32 | 100.33,97.79 C10.1 UC3.32 | C1.1 69.85,12.7
  Bottom 0.406: IC3.6 36.51,30.48 33.02,33.97 33.02,41.27 26.67,47.62 IC8.9 IC8.10 | IC8.12 IC8.13 IC8.14 | IC8.1 IC8.2 | UC4.31 UC4.32
  Bottom 0.813: C4.1 IC4.16 | C3.1 IC3.16 | C7.1 IC8.14 | C2.1 IC2.16 | C1.1 IC1.24 | VCC1.2 136.84,12.06 129.54,12.06 C6.1
/ALUCARRYIN
  Bottom 0.406: JP9.2 78.42,5.71 89.53,16.83 97.16,16.83 102.55,22.23 102.55,52.07 100.65,53.98 UC3.17
/ALUHI2MEM  (via drill 0.61 pad 1.27)
  Top 0.406: IC2.9 v43.81,55.24 | v112.39,44.45 101.6,55.24 v91.76,55.24 | v109.86,15.56 111.76,17.46 111.76,27.62 113.35,29.21 IC5.5
  Bottom 0.406: JP10.25 103.82,15.56 v109.86,15.56 | IC5.5 112.39,31.11 v112.39,44.45 | v43.81,55.24 v91.76,55.24
/ALULO2MEM  (via drill 0.61 pad 1.27)
  Top 0.406: IC2.10 45.72,34.92 v45.72,52.7 | v111.12,40.01 101.28,49.85 99.38,49.85 96.52,52.7 v92.71,52.7
  Bottom 0.406: v45.72,52.7 v92.71,52.7 | JP10.29 93.98,10.79 96.2,10.79 103.19,17.78 115.57,17.78 116.2,18.41 116.2,24.77 IC5.4 111.12,29.84 v111.12,40.01
/ALUSHR
  Bottom 0.406: JP9.1 78.42,8.26 88.9,18.73 96.52,18.73 100.65,22.86 100.65,49.53 93.66,56.52 UC3.15
/BUSIFCEN  (via drill 0.61 pad 1.27)
  Top 0.406: IC2.15 47.94,16.19 53.66,16.19 55.88,18.41 55.88,54.93 62.55,61.59 UC2.20 | v119.38,46.67 v103.19,62.87
  Bottom 0.406: IC8.4 21.59,43.81 22.86,45.09 22.86,58.1 25.08,60.33 42.23,60.33 44.77,57.78 61.59,57.78 65.41,61.59 UC2.20 75.25,61.59 76.52,62.87 v103.19,62.87 | JP10.5 121.92,13.02 120.02,14.92 120.02,46.04 v119.38,46.67
/CNT_SP
  Bottom 0.406: UC4.19 131.44,57.15 131.44,35.24 127.95,31.75 127.95,25.72 126.36,24.13 IC6.12
/CNTSP
  Top 0.406: JP10.3 128.59,12.38 128.59,23.81 IC6.11
/ENA
  Bottom 0.406: IC2.5 48.26,27.94 47.31,26.99 47.31,20.64 45.72,19.05 41.91,19.05 40.96,18.1 40.96,14.29 35.56,8.89 JP9.33
/ENABUS
  Bottom 0.406: IC3.13 29.84,25.4 31.11,24.13 31.11,13.97 26.67,9.53 26.67,4.45 28.89,2.22 98.11,2.22 JP10.22
/ENALU  (via drill 0.61 pad 1.27)
  Top 0.406: JP9.39 29.21,6.99 29.21,4.45 32.07,1.59 149.54,1.59 155.26,7.3 v155.26,22.23 | v151.76,22.23 138.11,22.23 136.21,24.13 IC6.3
  Bottom 0.406: v155.26,22.23 v151.76,22.23
/ENDP
  Bottom 0.406: JP9.44 20.64,3.49 16.51,3.49 13.97,6.03 13.97,9.21 10.79,12.38 10.79,30.48 12.06,31.75 20.64,31.75 21.91,30.48 IC4.6
/ENIPTR  (via drill 0.61 pad 1.27)
  Top 0.406: v33.34,27.94 IC3.12
  Bottom 0.406: JP9.38 31.75,6.99 31.75,8.89 36.51,13.65 36.51,15.56 34.61,17.46 34.61,24.45 33.34,25.72 v33.34,27.94
/ENLMDR
  Bottom 0.406: JP9.34 36.83,6.99 36.83,8.89 41.27,13.34 45.09,13.34 48.26,16.51 48.26,24.45 49.21,25.4 IC2.4
/ENMAR
  Bottom 0.406: JP9.48 17.78,6.35 19.05,7.62 19.05,10.16 20.64,11.75 20.64,13.65 24.45,17.46 24.45,24.13 23.18,25.4 IC4.4
/ENMEM  (via drill 0.61 pad 1.27)
  Top 0.406: v132.72,10.16 v132.72,13.97
  Bottom 0.406: JP10.16 110.49,4.45 128.91,4.45 132.72,8.26 v132.72,10.16 | IC6.6 131.76,31.75 130.49,30.48 130.49,18.41 132.72,16.19 v132.72,13.97
/ENMSW  (via drill 0.61 pad 1.27)
  Top 0.406: v32.38,22.86 IC3.14
  Bottom 0.406: JP9.40 29.21,6.99 29.21,8.89 32.38,12.06 v32.38,22.86
/ENPC
  Bottom 0.406: JP9.42 22.23,2.54 16.19,2.54 13.02,5.71 13.02,8.89 9.84,12.06 9.84,32.7 11.43,34.29 20.64,34.29 21.91,33.02 IC4.7
/ENPPC
  Bottom 0.406: JP9.37 30.48,8.89 35.56,13.97 35.56,15.24 33.66,17.14 33.66,24.13 31.43,26.35 31.43,29.21 30.16,30.48 IC3.11
/ENRMDR
  Bottom 0.406: IC3.15 28.57,20.32 27.3,19.05 27.3,16.19 25.4,14.29 JP9.41
/ENSP
  Bottom 0.406: JP9.46 21.59,6.99 21.59,13.34 25.4,17.14 25.4,25.72 23.18,27.94 IC4.5
/ENX
  Bottom 0.406: JP9.36 34.29,6.99 34.29,8.89 40.01,14.61 40.01,18.41 41.59,20 41.59,20.95 42.23,21.59 45.72,21.59 46.35,22.23 46.35,28.89 47.94,30.48 IC2.6
/ENY
  Bottom 0.406: JP9.35 33.02,8.89 39.05,14.92 39.05,18.73 40.64,20.32 40.64,22.54 41.59,23.5 41.59,30.8 42.55,31.75 49.85,31.75 51.12,33.02 IC2.7
/INC_MAR  (via drill 0.61 pad 1.27)
  Top 0.406: v149.22,3.81 147.96,2.54 41.27,2.54 JP9.32
  Bottom 0.406: UC4.20 137.79,57.15 137.79,43.18 149.22,31.75 v149.22,3.81
/INC_PC
  Bottom 0.406: UC4.21 131.76,64.14 130.49,62.87 130.49,35.88 126.36,31.75 IC6.9
/INCPC
  Bottom 0.406: JP10.1 127,12.06 122.87,16.19 122.87,32.07 125.09,34.29 IC6.8
/LATCH_I
  Bottom 0.406: JP9.47 12.7,13.34 12.7,26.67 13.97,27.94 IC4.12
/LATCH_NONE
  Bottom 0.406: IC8.5 24.13,39.37 22.54,37.78 16.51,37.78 14.61,35.88 IC4.9
/LATCH_S
  Bottom 0.406: JP9.45 20.32,7.62 19.05,6.35 19.05,5.08 18.41,4.45 17.14,4.45 14.92,6.67 14.92,9.53 11.75,12.7 11.75,29.21 13.02,30.48 IC4.11
/LATCHFLAGS  (via drill 0.61 pad 1.27)
  Top 0.406: JP10.12 113.03,6.99 103.5,6.99 102.87,6.35 102.87,4.76 101.92,3.81 45.4,3.81 44.45,4.76 44.45,9.53 42.55,11.43 v17.46,11.43
  Bottom 0.406: v17.46,11.43 17.46,17.46 IC4.15
/LDA
  Bottom 0.406: JP9.14 62.23,6.99 62.23,13.02 62.87,13.65 62.87,32.07 65.09,34.29 93.98,34.29 R6.2
/LDAHI
  Bottom 0.406: JP9.11 63.5,13.02 63.82,13.34 63.82,30.48 65.09,31.75 93.98,31.75 R5.2
/LDALO
  Bottom 0.406: JP9.12 64.77,6.99 64.77,27.94 66.04,29.21 93.98,29.21 R4.2
/LDDP
  Bottom 0.406: JP9.22 52.07,6.99 52.07,12.06 56.2,16.19 56.2,39.69 R14.2
/LDMAR
  Bottom 0.406: JP9.23 48.26,10.79 54.29,16.83 54.29,42.86 R12.2
/LDMARHI
  Bottom 0.406: JP9.17 55.88,12.06 59.05,15.24 59.05,34.61 61.91,37.47 61.91,45.4 63.5,46.99 93.98,46.99 R11.2
/LDMARLO
  Bottom 0.406: JP9.18 57.15,6.99 57.15,12.06 60.01,14.92 60.01,34.29 62.87,37.15 62.87,43.81 63.5,44.45 93.98,44.45 R10.2
/LDMDR
  Bottom 0.406: R3.2 93.98,26.67 66.99,26.67 65.72,25.4 65.72,8.57 JP9.9
/LDMDRHI
  Bottom 0.406: JP9.10 67.31,6.99 67.31,8.89 66.67,9.53 66.67,22.86 67.94,24.13 93.98,24.13 R2.2
/LDMDRLO
  Bottom 0.406: JP9.7 68.58,8.89 67.63,9.84 67.63,20.95 68.26,21.59 93.98,21.59 R1.2
/LDMEM  (via drill 0.61 pad 1.27)
  Top 0.406: R9.2 98.42,37.47 98.42,24.13 104.46,18.1 v104.46,14.29
  Bottom 0.406: v104.46,14.29 109.22,9.21 JP10.15
/LDMSW
  Bottom 0.406: JP9.20 54.61,6.99 54.61,12.06 58.1,15.56 58.1,36.51 R16.2
/LDPC
  Bottom 0.406: JP9.19 53.34,12.06 57.15,15.88 57.15,38.1 R15.2
/LDSP
  Bottom 0.406: JP9.21 50.8,12.06 55.24,16.51 55.24,41.27 R13.2
/LDX
  Bottom 0.406: JP9.13 60.96,13.34 61.91,14.29 61.91,32.38 66.36,36.83 93.98,36.83 R7.2
/LDY
  Bottom 0.406: JP9.16 59.69,6.99 59.69,13.34 60.96,14.61 60.96,32.7 64.77,36.51 64.77,38.1 66.04,39.37 93.98,39.37 R8.2
/LOAD_IR  (via drill 0.61 pad 1.27)
  Top 0.406: UC2.14 56.2,59.05 60.01,62.87 72.71,62.87 77.15,58.42 77.15,19.68 81.92,14.92 100.65,14.92 v102.87,12.7
  Bottom 0.406: v102.87,12.7 102.87,11.75 100.33,9.21 100.33,7.62 99.69,6.99 97.79,6.99 JP10.26
/MEM2ALUHI  (via drill 0.61 pad 1.27)
  Top 0.406: v47.31,51.44 47.31,33.97 IC2.11 | v116.2,16.83 116.2,19.68 IC5.2 | v109.86,38.1 96.52,51.44 v91.44,51.44
  Bottom 0.406: v47.31,51.44 v91.44,51.44 | JP10.27 95.57,9.84 96.52,9.84 103.5,16.83 v116.2,16.83 | IC5.2 109.86,26.04 v109.86,38.1
/MEM2ALULO  (via drill 0.61 pad 1.27)
  Top 0.406: IC2.12 42.86,27.94 41.59,29.21 v41.59,50.16 | v108.58,36.2 94.61,50.16 v90.17,50.16
  Bottom 0.406: v41.59,50.16 v90.17,50.16 | JP10.31 92.39,11.75 95.89,11.75 104.46,20.32 109.86,20.32 111.12,19.05 IC5.1 108.58,25.08 v108.58,36.2
ADDRBUS0
  Top 0.406: IC4.2 21.27,20.32 17.78,23.81 17.78,46.99 17.78,48.58 17.78,50.8 16.51,52.07 16.51,56.83 18.73,59.05 UC1.14
ADDRBUS1
  Top 0.406: IC4.3 21.27,22.86 20.32,23.81 20.32,43.81 21.91,45.4 24.13,45.4 25.4,46.67 25.4,54.61 23.5,56.52 UC1.15
ALUMODE
  Bottom 0.406: JP9.3 74.93,6.99 78.42,6.99 89.22,17.78 96.84,17.78 101.6,22.54 101.6,49.85 98.42,53.02 98.42,55.56 99.38,56.52 UC3.18
ALUOP0
  Bottom 0.406: JP9.4 74.93,4.45 78.42,4.45 89.85,15.88 97.47,15.88 103.5,21.91 103.5,56.52 100.97,59.05 UC3.19
ALUOP1
  Bottom 0.406: JP9.6 73.34,3.49 78.74,3.49 90.17,14.92 97.79,14.92 104.46,21.59 104.46,58.74 101.6,61.59 UC3.20
ALUOP2  (via drill 0.61 pad 1.27)
  Top 0.406: UC3.21 99.06,62.87 82.87,62.87 80.01,60.01 v80.01,19.68
  Bottom 0.406: v80.01,19.68 80.01,17.14 JP9.5
ALUOP3  (via drill 0.61 pad 1.27)
  Top 0.406: v78.42,20.32 78.42,58.74 71.75,65.41 59.69,65.41 55.88,61.59 UC2.13
  Bottom 0.406: JP9.8 69.85,6.99 69.85,9.21 78.42,17.78 v78.42,20.32
BUSCLKA  (via drill 0.61 pad 1.27)
  Top 0.406: IC1.18 71.12,35.56 75.56,31.11 75.56,20 81.92,13.65 v91.12,13.65 | v87,9.53 87.31,9.84 97.47,9.84 JP10.23
  Bottom 0.406: v91.12,13.65 v87,9.53
BUSIFCMODE0  (via drill 0.61 pad 1.27)
  Top 0.406: IC4.14 12.38,25.08 12.38,51.44 14.29,53.34 14.29,59.69 17.46,62.87 v24.45,62.87 | IC2.14 46.04,22.86 49.85,19.05 53.98,19.05 54.93,20 54.93,56.52 53.66,57.78 49.85,57.78 v44.77,62.87
  Bottom 0.406: UC2.21 66.04,62.87 v44.77,62.87 v24.45,62.87
BUSIFCMODE1
  Top 0.406: IC4.13 15.56,25.4 16.83,26.67 16.83,36.83 15.24,38.42 15.24,46.99 15.24,47.62 15.24,58.42 18.41,61.59 UC1.13 22.54,61.59 40.64,43.5 40.64,27.3 42.55,25.4 IC2.13
CLBUS0
  Top 0.406: IC2.2 50.8,20.32 48.58,22.54 48.58,52.39 39.37,61.59 UC1.20
CLBUS1
  Top 0.406: IC2.3 50.8,22.86 49.53,24.13 49.53,52.7 38.1,64.14 UC1.21
CLK0D  (via drill 0.61 pad 1.27)
  Top 0.406: v134.94,7.62 136.84,9.53 136.84,18.41 133.67,21.59 IC6.2
  Bottom 0.406: IC6.2 132.72,21.59 131.44,22.86 131.44,27.62 132.72,29.21 IC6.5 | JP10.17 107.95,6.99 107.95,4.45 108.9,3.49 130.81,3.49 v134.94,7.62
CNT0
  Bottom 0.406: UC4.8 109.22,74.3 107.95,75.56 92.71,75.56 91.44,74.3 UC3.8 76.52,74.3 75.25,75.56 60.96,75.56 59.69,74.3 UC2.8 43.81,74.3 42.55,75.56 27.94,75.56 26.67,74.3 UC1.8 JP8.1
CNT1
  Bottom 0.406: UC4.7 109.22,76.83 107.95,78.11 92.71,78.11 91.44,76.83 UC3.7 76.52,76.83 75.25,78.11 60.96,78.11 59.69,76.83 UC2.7 43.81,76.83 42.55,78.11 27.94,78.11 26.67,76.83 UC1.7 JP8.2
CNT2
  Bottom 0.406: UC4.6 109.22,79.38 107.95,80.64 92.71,80.64 91.44,79.38 UC3.6 76.52,79.38 75.25,80.64 60.96,80.64 59.69,79.38 UC2.6 43.81,79.38 42.55,80.64 27.94,80.64 26.67,79.38 UC1.6 JP8.3
CNT3
  Bottom 0.406: UC4.5 109.22,81.92 107.95,83.19 92.71,83.19 91.44,81.92 UC3.5 76.52,81.92 75.25,83.19 60.96,83.19 59.69,81.92 UC2.5 43.81,81.92 42.55,83.19 27.94,83.19 26.67,81.92 UC1.5 JP8.4
CNT4
  Top 0.406: UC1.27 30.48,83.19 14.29,83.19 JP8.5
  Bottom 0.406: UC4.27 125.73,79.38 124.46,78.11 109.22,78.11 107.95,79.38 UC3.27 92.71,79.38 91.44,78.11 76.52,78.11 75.25,79.38 UC2.27 60.96,79.38 59.69,78.11 43.81,78.11 42.55,79.38 UC1.27
CRBUS0
  Bottom 0.406: IC3.1 39.69,20.64 39.69,23.18 40.64,24.13 40.64,37.47 32.7,45.4 32.7,52.7 33.97,53.98 UC1.17
CRBUS1
  Bottom 0.406: IC3.2 38.73,22.23 38.73,23.5 39.69,24.45 39.69,37.15 31.75,45.09 31.75,53.98 UC1.18
CRBUS2
  Bottom 0.406: IC3.3 38.73,24.77 38.73,36.83 30.8,44.77 30.8,55.56 UC1.19
FAULT  (via drill 0.61 pad 1.27)
  Top 0.406: v73.98,41.91 66.36,41.91 65.41,40.96 65.41,37.47 IC1.19 | IC6.10 120.65,29.21 119.38,30.48 103.82,30.48 99.38,34.92 99.38,40.64 v98.11,41.91 | JP10.28 95.25,6.99 99.69,6.99 100.33,7.62 100.33,9.21 100.97,9.84 124.14,9.84 127.64,13.34 127.64,19.68 IC6.13
  Bottom 0.406: IC6.13 123.83,23.5 123.83,27.3 IC6.10 | v98.11,41.91 v73.98,41.91
FC
  Bottom 0.406: UC1.9 26.67,71.75 27.94,73.03 42.55,73.03 43.81,71.75 UC2.9 59.69,71.75 60.96,73.03 75.25,73.03 76.52,71.75 UC3.9 91.44,71.75 92.71,73.03 107.95,73.03 109.22,71.75 UC4.9 121.92,68.26 121.92,15.88 125.73,12.06 125.73,6.99 JP10.2
FN
  Bottom 0.406: UC1.11 26.67,66.67 27.94,67.94 42.55,67.94 43.81,66.67 UC2.11 59.69,66.67 60.96,67.94 75.25,67.94 76.52,66.67 UC3.11 91.44,66.67 92.71,67.94 107.95,67.94 109.22,66.67 UC4.11 118.75,66.67 120.02,65.41 120.02,53.02 116.52,49.53 116.52,46.04 119.06,43.5 119.06,14.29 120.65,12.7 120.65,6.99 JP10.6
FV
  Bottom 0.406: UC1.12 26.67,64.14 27.94,65.41 42.55,65.41 43.81,64.14 UC2.12 59.69,64.14 60.96,65.41 75.25,65.41 76.52,64.14 UC3.12 91.44,64.14 92.71,65.41 107.95,65.41 109.22,64.14 UC4.12 117.16,64.14 114.62,61.59 114.62,46.67 118.11,43.18 118.11,6.99 JP10.8
FZ
  Bottom 0.406: UC1.10 26.67,69.22 27.94,70.48 42.55,70.48 43.81,69.22 UC2.10 59.69,69.22 60.96,70.48 75.25,70.48 76.52,69.22 UC3.10 91.44,69.22 92.71,70.48 107.95,70.48 109.22,69.22 UC4.10 120.97,66.67 120.97,15.56 123.19,13.34 123.19,6.99 JP10.4
GND
  Bottom 0.813: C2.2 51.44,17.14 IC2.1
  pour Top (isolate 0.61): 0,100.01 160.02,100.01 160.02,0 0,0
  pour Bottom (isolate 0.61): 0,100.01 160.02,100.01 160.02,0 0,0
LOAD0  (via drill 0.61 pad 1.27)
  Top 0.406: IC1.23 60.96,31.75 v60.96,56.52
  Bottom 0.406: v60.96,56.52 UC2.15
LOAD1
  Top 0.406: IC1.22 61.91,33.34 61.91,50.48 65.41,53.98 UC2.17
LOAD2
  Top 0.406: IC1.21 63.5,34.29 63.5,49.53 65.09,51.12 67.63,51.12 69.22,52.7 69.22,55.24 67.94,56.52 UC2.18
LOAD3
  Top 0.406: UC2.19 70.17,56.2 70.17,52.39 67.94,50.16 65.41,50.16 64.45,49.21 64.45,35.88 IC1.20
LOAD_FLAGS0  (via drill 0.61 pad 1.27)
  Top 0.406: UC3.13 81.6,58.1 v81.6,19.05 | v75.56,10.16 50.48,10.16 49.53,9.21 49.53,6.99 JP9.24
  Bottom 0.406: v81.6,19.05 81.6,16.19 v75.56,10.16
LOAD_FLAGS1  (via drill 0.61 pad 1.27)
  Top 0.406: UC3.14 83.19,57.15 v83.19,18.41 | v78.42,10.48 77.47,11.43 48.9,11.43 46.99,9.53 46.99,6.99 JP9.26
  Bottom 0.406: v83.19,18.41 83.19,15.24 v78.42,10.48
MDRLDINHBT
  Bottom 0.406: JP9.43 22.86,13.02 26.35,16.51 26.35,40.96 IC8.6
MEMSEG
  Top 0.406: JP10.14 113.03,4.45 146.05,4.45 147.96,6.35 151.76,6.35 153.03,7.62 153.03,34.29 UC4.17
N$1
  Bottom 0.406: IC1.16 R15.1
N$8
  Top 0.406: IC6.1 129.54,22.86 129.54,26.35 127.95,27.94 118.11,27.94 IC5.3
N$15
  Top 0.406: IC6.4 129.54,30.48 120.97,30.48 119.7,31.75 IC5.6
N$31
  Bottom 0.406: R1.1 IC1.1
N$33
  Bottom 0.406: R2.1 IC1.2
N$34
  Bottom 0.406: R3.1 IC1.3
N$35
  Bottom 0.406: R4.1 IC1.4
N$36
  Bottom 0.406: R5.1 IC1.5
N$37
  Bottom 0.406: R6.1 IC1.6
N$38
  Bottom 0.406: R7.1 IC1.7
N$39
  Bottom 0.406: IC1.8 R8.1
N$40
  Bottom 0.406: R9.1 IC1.9
N$41
  Bottom 0.406: R10.1 IC1.10
N$42
  Bottom 0.406: IC1.11 R11.1
N$43
  Bottom 0.406: IC1.13 R12.1
N$44
  Bottom 0.406: IC1.14 R13.1
N$45
  Bottom 0.406: IC1.15 R14.1
N$56
  Bottom 0.406: IC1.17 R16.1
OP0
  Bottom 0.406: UC1.26 42.55,76.83 43.81,75.56 59.69,75.56 60.96,76.83 UC2.26 75.25,76.83 76.52,75.56 91.44,75.56 92.71,76.83 UC3.26 107.95,76.83 109.22,75.56 124.46,75.56 125.73,76.83 UC4.26 140.97,76.83 143.51,74.3 143.51,48.9 152.72,39.69 JP7.9
OP1
  Top 0.406: UC3.23 101.6,70.48 132.08,70.48 UC4.23 139.7,69.22 144.78,64.14 144.78,50.16 152.72,42.23 JP7.8
  Bottom 0.406: UC1.23 42.55,69.22 43.81,67.94 59.69,67.94 60.96,69.22 UC2.23 75.25,69.22 76.52,67.94 91.44,67.94 92.71,69.22 UC3.23
OP2
  Top 0.406: UC4.25 142.24,74.3 146.05,70.48 146.05,51.44 152.72,44.77 JP7.7
  Bottom 0.406: UC4.25 125.73,74.3 124.46,73.03 109.22,73.03 107.95,74.3 UC3.25 92.71,74.3 91.44,73.03 76.52,73.03 75.25,74.3 UC2.25 60.96,74.3 59.69,73.03 43.81,73.03 42.55,74.3 UC1.25
OP3
  Top 0.406: UC4.4 124.46,84.45 125.73,83.19 140.97,83.19 147.32,76.83 147.32,52.7 152.72,47.31 JP7.6
  Bottom 0.406: UC4.4 109.22,84.45 107.95,85.72 92.71,85.72 91.44,84.45 UC3.4 76.52,84.45 75.25,85.72 60.96,85.72 59.69,84.45 UC2.4 43.81,84.45 42.55,85.72 27.94,85.72 26.67,84.45 UC1.4
OP4
  Bottom 0.406: UC1.28 42.55,81.92 43.81,80.64 59.69,80.64 60.96,81.92 UC2.28 75.25,81.92 76.52,80.64 91.44,80.64 92.71,81.92 UC3.28 107.95,81.92 109.22,80.64 124.46,80.64 125.73,81.92 UC4.28 143.83,81.92 148.59,77.15 148.59,53.98 152.72,49.85 JP7.5
OP5
  Bottom 0.406: UC1.29 42.55,84.45 43.81,83.19 59.69,83.19 60.96,84.45 UC2.29 75.25,84.45 76.52,83.19 91.44,83.19 92.71,84.45 UC3.29 107.95,84.45 109.22,83.19 124.46,83.19 125.73,84.45 UC4.29 142.88,84.45 149.86,77.47 149.86,55.24 152.72,52.39 JP7.4
OP6
  Top 0.406: JP7.3 152.72,54.93 151.13,56.52 151.13,77.79 143.19,85.72 125.73,85.72 124.46,87 UC4.3
  Bottom 0.406: UC4.3 109.22,87 107.95,88.27 92.71,88.27 91.44,87 UC3.3 76.52,87 75.25,88.27 60.96,88.27 59.69,87 UC2.3 43.81,87 42.55,88.27 27.94,88.27 26.67,87 UC1.3
OP7
  Bottom 0.406: UC1.2 26.67,89.53 27.94,90.81 42.55,90.81 43.81,89.53 UC2.2 59.69,89.53 60.96,90.81 75.25,90.81 76.52,89.53 UC3.2 91.44,89.53 92.71,90.81 107.95,90.81 109.22,89.53 UC4.2 124.46,89.53 125.73,88.27 143.83,88.27 155.57,76.52 155.57,58.74 154.31,57.47 JP7.2
OP8
  Bottom 0.406: UC1.30 42.55,87 43.81,85.72 59.69,85.72 60.96,87 UC2.30 75.25,87 76.52,85.72 91.44,85.72 92.71,87 UC3.30 107.95,87 109.22,85.72 124.46,85.72 125.73,87 UC4.30 143.51,87 153.35,77.15 JP7.1
PROT  (via drill 0.61 pad 1.27)
  Top 0.406: v141.29,38.1 122.87,56.52 UC4.15
  Bottom 0.406: JP10.21 102.87,6.99 102.87,3.81 104.14,2.54 144.15,2.54 148.27,6.67 148.27,31.11 v141.29,38.1
SP_DIR
  Top 0.406: JP10.20 106.36,3.49 146.69,3.49 148.59,5.4 152.08,5.4 153.99,7.3 153.99,34.92 135.89,53.02 135.89,54.93 134.3,56.52 UC4.18

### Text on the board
Top: #2
_tsilk: VCC2 | GND1 | UC1 | UC2 | UC3 | UC4 | AM29F020P | AM29F020P | AM29F020P | AM29F020P | JP3 | JP8 | JP7 | 74LS08N | IC8 | JP4 | JP2 | 74154N | 70 | 74LS00N | 74LS32N | 74LS139N | 74LS138N | 74LS139N | IC1 | IC5 | IC6 | IC4 | IC3 | IC2 | GND2 | VCC1 | 10u | JP9 | JP10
